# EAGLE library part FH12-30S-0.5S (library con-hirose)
0.5mm Pitch Connectors For FPC/FFC Source: Data sheet
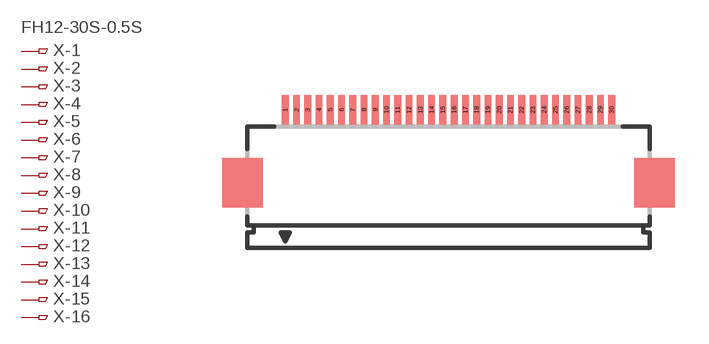
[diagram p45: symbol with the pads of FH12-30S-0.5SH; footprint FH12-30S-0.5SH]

Designator prefix X; gates -1=PINV -2=PIN -3=PIN -4=PIN -5=PIN -6=PIN -7=PIN -8=PIN -9=PIN -10=PIN -11=PIN -12=PIN -13=PIN -14=PIN -15=PIN -16=PIN -17=PIN -18=PIN -19=PIN -20=PIN -21=PIN -22=PIN -23=PIN -24=PIN -25=PIN -26=PIN -27=PIN -28=PIN -29=PIN -30=PIN

## FH12-30S-0.5SH (MPN: FH12-30S-0.5SH(55); OC_FARNELL: 1324555; OC_NEWARK: 34M6176)  [FH12-30S-0.5SH]
1  -1:1  pas
2  -2:1  pas
3  -3:1  pas
4  -4:1  pas
5  -5:1  pas
6  -6:1  pas
7  -7:1  pas
8  -8:1  pas
9  -9:1  pas
10  -10:1  pas
11  -11:1  pas
12  -12:1  pas
13  -13:1  pas
14  -14:1  pas
15  -15:1  pas
16  -16:1  pas
17  -17:1  pas
18  -18:1  pas
19  -19:1  pas
20  -20:1  pas
21  -21:1  pas
22  -22:1  pas
23  -23:1  pas
24  -24:1  pas
25  -25:1  pas
26  -26:1  pas
27  -27:1  pas
28  -28:1  pas
29  -29:1  pas
30  -30:1  pas

## Footprint FH12-30S-0.5SH (pad centres in mm)
0.5mm Pitch Connectors For FPC/FFC Source: Data sheet
smd 0.3 x 1.3: 1 -7.25,3.25; 2 -6.75,3.25; 3 -6.25,3.25; 4 -5.75,3.25; 5 -5.25,3.25; 6 -4.75,3.25; 7 -4.25,3.25; 8 -3.75,3.25; 9 -3.25,3.25; 10 -2.75,3.25; 11 -2.25,3.25; 12 -1.75,3.25; 13 -1.25,3.25; 14 -0.75,3.25; 15 -0.25,3.25; 16 0.25,3.25; 17 0.75,3.25; 18 1.25,3.25; 19 1.75,3.25; 20 2.25,3.25; 21 2.75,3.25; 22 3.25,3.25; 23 3.75,3.25; 24 4.25,3.25; 25 4.75,3.25; 26 5.25,3.25; 27 5.75,3.25; 28 6.25,3.25; 29 6.75,3.25; 30 7.25,3.25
